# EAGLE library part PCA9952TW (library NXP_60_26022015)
16-channel Fm+ I2C-bus 57 mA constant current LED driver The PCA9952 and PCA9955 are I2 C-bus controlled 16-channel constant current LED driver optimized for dimming and blinking 57 mA Red/Green/Blue/Amber (RGBA) LEDs in amusement products. Each LEDn output has its own 8-bit resolution (256 steps) fixed frequency individual PWM controller that operates at 31.25 kHz with a duty cycle that is adjustable from 0 % to 99.6 % to allow the LED to be set to a specific brightness value. An additional 8-bit resolution (256 steps) group PWM controller has both a fixed frequency of 122 Hz and an adjustable frequency between 15 Hz to once every 16.8 seconds with a duty cycle that is adjustable from 0 % to 99.6 % that is used to either dim or blink all LEDs with the same value. Each LEDn output can be off, on (no PWM control), set at its individual PWM controller value or at both individual and group PWM controller values. The PCA9952 and PCA9955 operate with a supply voltage range of 3 V to 5.5 V and the constant current sink LEDn outputs allow up to 40 V for the LED supply. The output peak current is adjustable with an 8-bit linear DAC from 225 uA to 57 mA. These devices have built-in open, short load and overtemperature detection circuitry. The error information from the corresponding register can be read via the I2 C-bus. Additionally, a thermal shutdown feature protects the device when internal junction temperature exceeds the limit allowed for the process. The PCA9952 and PCA9955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
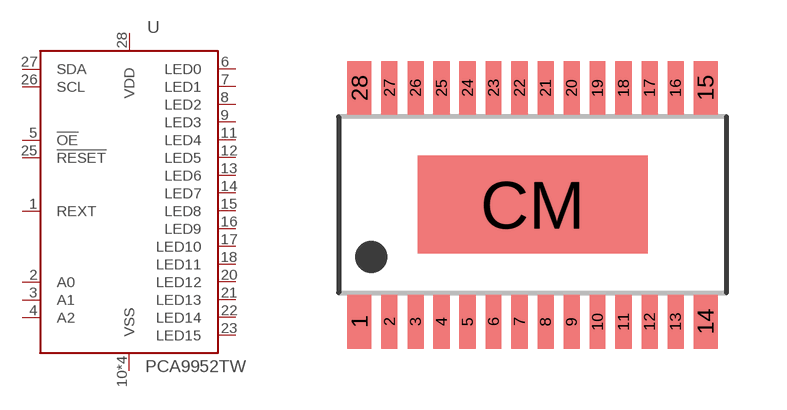
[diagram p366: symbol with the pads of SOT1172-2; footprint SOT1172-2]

Designator prefix U

## PCA9952TW, PCA9952TW/Q900  [SOT1172-2]
1  REXT  pas
2  A0  in
3  A1  in
4  A2  in
5  !OE  in
6  LED0  out
7  LED1  out
8  LED2  out
9  LED3  out
10  VSS  pwr
11  LED4  out
12  LED5  out
13  LED6  out
14  LED7  out
15  LED8  out
16  LED9  out
17  LED10  out
18  LED11  out
19  VSS  pwr
20  LED12  out
21  LED13  out
22  LED14  out
23  LED15  out
24  VSS  pwr
25  !RESET!  in
26  SCL
27  SDA
28  VDD  pwr
CM  VSS  pwr

## Footprint SOT1172-2 (pad centres in mm)
SOT1172-2 HTSSOP28: plastic thermal enhanced thin shrink small outline package; 28 leads; body width 4.4 mm; lead pitch 0.65 mm; exposed die pad JEDEC: MO-153 IEC: -- JEITA: --date: 2013-08-05
smd 0.6 x 1.35: 1 -4.325,-2.925; 14 4.325,-2.925; 15 4.325,2.925; 28 -4.325,2.925
smd 0.4 x 1.35: 2 -3.575,-2.925; 3 -2.925,-2.925; 4 -2.275,-2.925; 5 -1.625,-2.925; 6 -0.975,-2.925; 7 -0.325,-2.925; 8 0.325,-2.925; 9 0.975,-2.925; 10 1.625,-2.925; 11 2.275,-2.925; 12 2.925,-2.925; 13 3.575,-2.925; 16 3.575,2.925; 17 2.925,2.925; 18 2.275,2.925; 19 1.625,2.925; 20 0.975,2.925; 21 0.325,2.925; 22 -0.325,2.925; 23 -0.975,2.925; 24 -1.625,2.925; 25 -2.275,2.925; 26 -2.925,2.925; 27 -3.575,2.925
smd 5.75 x 2.45: CM 0,0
